FUNCTION FC 22 : VOID
TITLE =USCITE E COMANDI CESOIA
VERSION : 0.1

BEGIN
NETWORK
TITLE =DISCESA MANUALE CESOIA
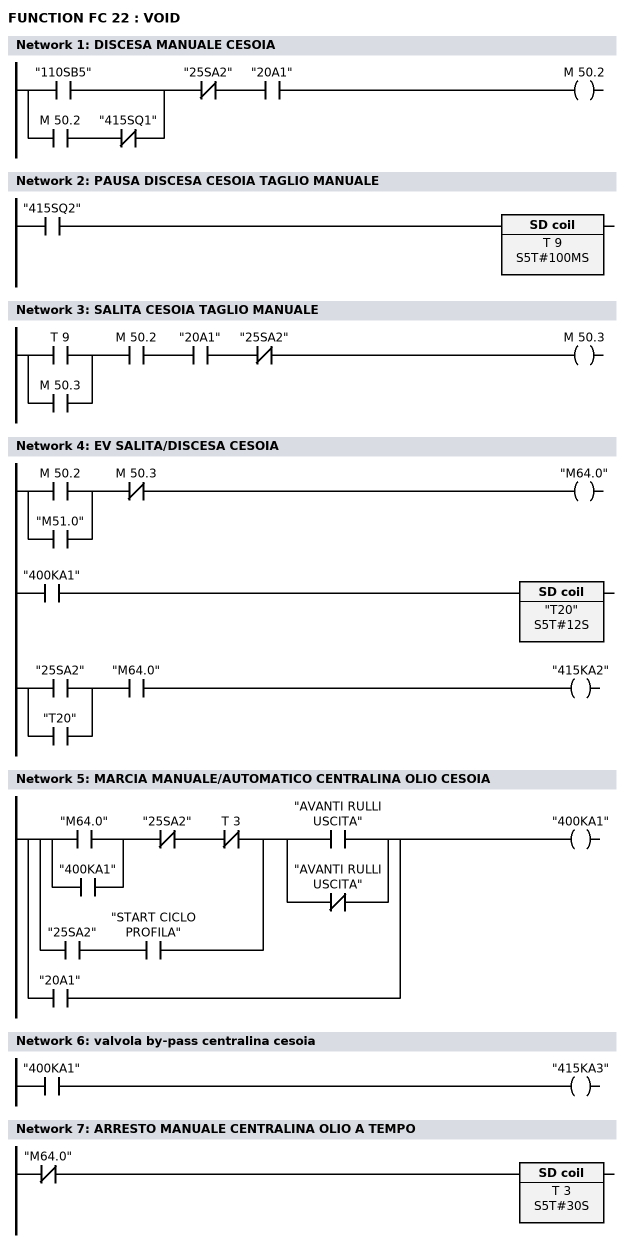
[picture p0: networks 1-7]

      U     "110SB5";
      O(    ;
      U     M     50.2;
      UN    "415SQ1";
      )     ;
      UN    "25SA2";
      U     "20A1";
      =     M     50.2;
NETWORK
TITLE =PAUSA DISCESA CESOIA TAGLIO MANUALE

      U     "415SQ2";
      L     S5T#100MS;
      SE    T      9;
NETWORK
TITLE =SALITA CESOIA TAGLIO MANUALE

      U(    ;
      O     T      9;
      O     M     50.3;
      )     ;
//      UN    "415SQ1"
      U     M     50.2;
      U     "20A1";
      UN    "25SA2";
      =     M     50.3;
NETWORK
TITLE =EV SALITA/DISCESA CESOIA

      U(    ;
      O     M     50.2;
      O     "M51.0";
      )     ;
      UN    M     50.3;
      =     "M64.0";

      U     "400KA1";
      L     S5T#12S;
      SE    "T20";

      U     "25SA2";
      O     "T20";
      U     "M64.0";
      =     "415KA2";
NETWORK
TITLE =MARCIA MANUALE/AUTOMATICO CENTRALINA OLIO CESOIA

      U(    ;
      U(    ;
      O     "M64.0";
      O     "400KA1";
      )     ;
      UN    "25SA2";
      UN    T      3;
      O     ;
      U     "25SA2";
      U     "START CICLO PROFILA";
      )     ;
      U(    ;
      O     "AVANTI RULLI USCITA";
      ON    "AVANTI RULLI USCITA";
      )     ;
      O     "20A1";
      =     "400KA1";
NETWORK
TITLE =valvola by-pass centralina cesoia

      U     "400KA1";
      =     "415KA3";
NETWORK
TITLE =ARRESTO MANUALE CENTRALINA OLIO A TEMPO

      UN    "M64.0";
      L     S5T#30S;
      SE    T      3;
END_FUNCTION

